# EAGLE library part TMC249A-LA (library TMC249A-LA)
High Current Microstep Stepper Motor Driver with sensorless stall detection, protection / diagnosis and SPI Interface, QFN32(7x7)
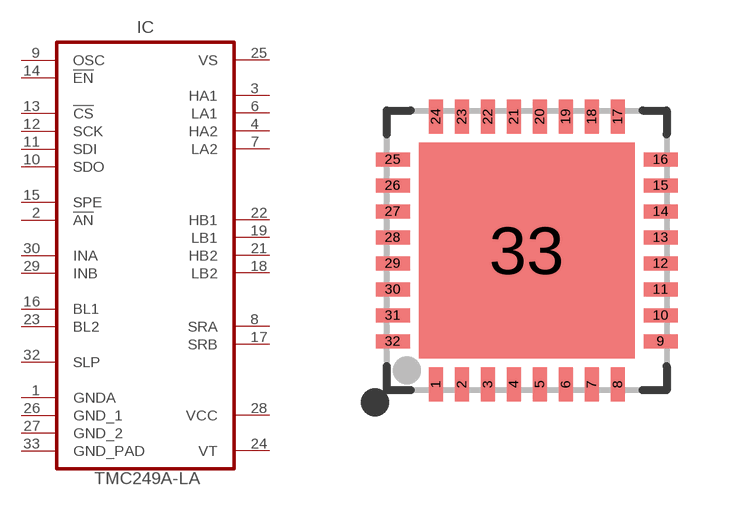
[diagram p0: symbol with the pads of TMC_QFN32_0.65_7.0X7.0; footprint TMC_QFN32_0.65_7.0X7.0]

Designator prefix IC

## TMC249A-LA (DATASHEET: http://www_trinamic_com/_scripts/download_php?file=_articles%2Fproducts%2Fintegrated-circuits%2Ftmc249%2F_datasheet%2FTMC249_datasheet_pdf; DESCRIPTION: High Current Microstep Stepper Motor Driver with sensorless stall detection, protection / diagnosis and SPI Interface, QFN32(7x7); DISTRIBUTOR1: Digikey; GEOMETRY_HEIGHT: 1mm; MANUFACTURER: TRINAMIC; ORDERCODE-DISTRI1: 1460-1041-ND; ORDERCODE-MANU1: TMC249A-LA; VALUE: TMC249A-LA)  [TMC_QFN32_0.65_7.0X7.0]
1  GNDA  pwr
2  !AN!  in
3  HA1  out
4  HA2  out
6  LA1  out
7  LA2  out
8  SRA  in
9  OSC
10  SDO  out
11  SDI  in
12  SCK  in
13  !CS!  in
14  !EN!  in
15  SPE  in
16  BL1  in
17  SRB  in
18  LB2  out
19  LB1  out
21  HB2  out
22  HB1  out
23  BL2  in
24  VT  pwr
25  VS  pwr
26  GND_1  pwr
27  GND_2  pwr
28  VCC  pwr
29  INB  in
30  INA  in
32  SLP  in
33  GND_PAD  pwr

## Footprint TMC_QFN32_0.65_7.0X7.0 (pad centres in mm)
smd 0.35 x 0.85: 1 -2.275,-3.35; 2 -1.625,-3.35; 3 -0.975,-3.35; 4 -0.325,-3.35; 5 0.325,-3.35; 6 0.975,-3.35; 7 1.625,-3.35; 8 2.275,-3.35; 17 2.275,3.35; 18 1.625,3.35; 19 0.975,3.35; 20 0.325,3.35; 21 -0.325,3.35; 22 -0.975,3.35; 23 -1.625,3.35; 24 -2.275,3.35
smd 0.85 x 0.35: 9 3.35,-2.275; 10 3.35,-1.625; 11 3.35,-0.975; 12 3.35,-0.325; 13 3.35,0.325; 14 3.35,0.975; 15 3.35,1.625; 16 3.35,2.275; 25 -3.35,2.275; 26 -3.35,1.625; 27 -3.35,0.975; 28 -3.35,0.325; 29 -3.35,-0.325; 30 -3.35,-0.975; 31 -3.35,-1.625; 32 -3.35,-2.275
smd 5.4 x 5.4: 33 0,0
